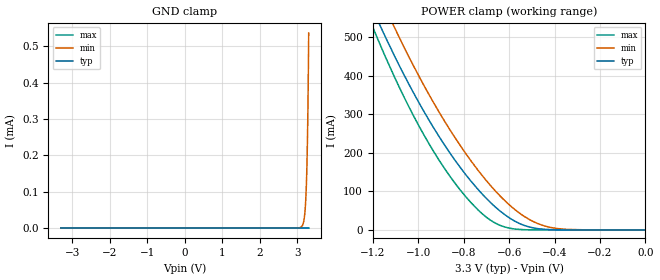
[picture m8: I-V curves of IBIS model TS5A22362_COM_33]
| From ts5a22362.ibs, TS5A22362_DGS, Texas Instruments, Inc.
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[Model]   TS5A22362_COM_33
Model_type  Terminator
| variable   typ   min   max
C_comp   158.70pF   114.52pF   195.75pF
| C_tri-state   158.70pF   114.52pF   195.75pF
[Temperature Range]   40   100   -40
| Ambient temperature   25   85   -40
[Voltage range]   3.3   3   3.6
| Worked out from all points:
|   POWER clamp passes 1 mA (typ) near -0.42 V on its own axis
[GND Clamp]
| TS5A22362_COM_33
|   Voltage   I(typ)   I(min)   I(max)
-3.3V     -7.587nA   -380.6nA   -3.915nA
3.1V      4.04nA     2.798uA    3.133nA
3.15V     4.109nA    11.39uA    3.187nA
3.185V    4.164nA    29.69uA    3.225nA
3.21V     4.214nA    57.69uA    3.252nA
3.235V    4.292nA    110uA      3.278nA
3.255V    4.404nA    181.7uA    3.3nA
3.27V     4.549nA    262.5uA    3.316nA
3.28V     4.698nA    334.2uA    3.327nA
3.285V    4.795nA    376.6uA    3.332nA
3.295V    5.05nA     477.2uA    3.343nA
3.3V      5.219nA    536.6uA    3.348nA
[POWER Clamp]
| TS5A22362_COM_33
|   Voltage   I(typ)   I(min)   I(max)
-3.3V     5.457A     5.491A     6.033A
-1.21V    586.1mA    663.4mA    541mA
-1.19V    559.5mA    636.3mA    512.3mA
-1.165V   527.1mA    603mA      477.4mA
-1.105V   452.5mA    526.3mA    397.8mA
-995mV    328.5mA    397.2mA    268mA
-870mV    208.1mA    269.1mA    147.4mA
-770mV    128.3mA    181.2mA    72.44mA
-670mV    64.66mA    107.5mA    20.89mA
-555mV    16.91mA    44mA       1.409mA
-445mV    1.761mA    10.61mA    34.89uA
0V        0A         0A         0A
